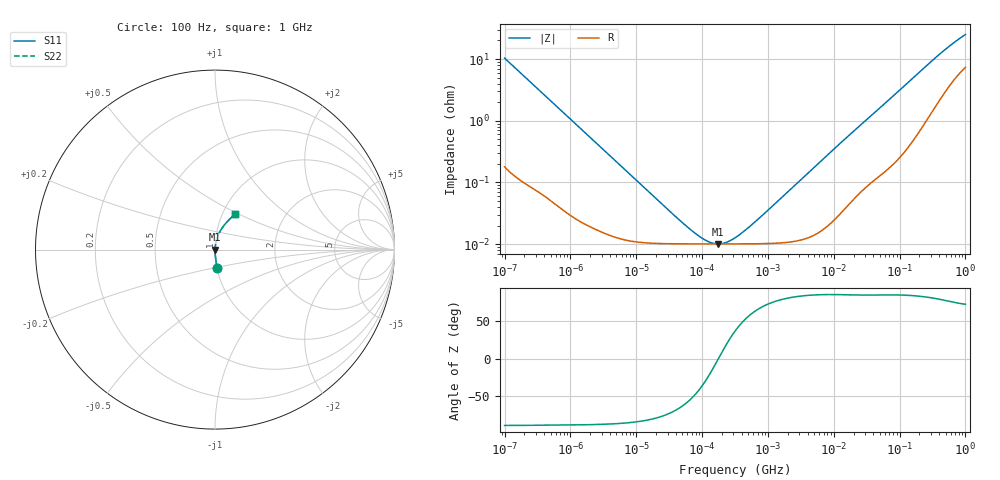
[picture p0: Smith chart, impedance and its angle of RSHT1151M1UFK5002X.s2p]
! RSHT1151M1UFK5002X  S-PARAMETER MODEL  (General Type)
! Model Generated by ELNA Corporation (http://www.ty-top.com)
! Version 1.0
! ELNA Control No.201201
! Copyright (c) 2020 ELNA CO.,LTD. All Rights Reserved.
! Products Name : CONDUCTIVE POLYMER HYBRID ALUMINUM ELECTROLYTIC CAPACITORS
! Characteristics :
!  Capacitance  :  150uF  ,  Rated voltage  :  50V
!  Operating Temp. Range  :  -55 to +105 degC  ,  Endurance  :  5000hr at 105 degC
!  Dimension D  :  10mm  ,  Dimension L  :  12.5mm
! Frequency Range : 100Hz - 1GHz
! External Node Assignments :
!  1  o---| |---o  2
# MHz S RI R 50
!Freq[MHz].  S11 Real  S11 Imag  S21 Real  S21 Imag  S12 Real  S12 Imag  S22 Real  S22 Imag
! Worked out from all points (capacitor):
!   401 points, 100 Hz to 1 GHz, reference 50 ohm
!   read as one part in series: C = 153 uF near 108 Hz
!   lowest |Z| = 10.1 mohm at 172.8 kHz (marker M1)
!   series resonance near 176.2 kHz, so ESL is about 5.3 nH
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0.0001  0.0124 -0.1021  0.9876 0.1021  0.9876 0.1021  0.0124 -0.1021
0.000113  0.0099 -0.0908  0.9901 0.0908  0.9901 0.0908  0.0099 -0.0908
0.000183  0.00424 -0.0565  0.9958 0.0565  0.9958 0.0565  0.00424 -0.0565
0.000309  0.00187 -0.0337  0.9981 0.0337  0.9981 0.0337  0.00187 -0.0337
0.001488  0.000276 -0.00717  0.9997 0.00717  0.9997 0.00717  0.000276 -0.00717
0.022131  0.000103 -0.000484  0.9999 0.000484  0.9999 0.000484  0.000103 -0.000484
0.051582  0.000101 -0.000193  0.9999 0.000193  0.9999 0.000193  0.000101 -0.000193
0.087096  0.000101 -9.44e-05  0.9999 9.44e-05  0.9999 9.44e-05  0.000101 -9.44e-05
0.12517  0.000101 -4.31e-05  0.9999 4.31e-05  0.9999 4.31e-05  0.000101 -4.31e-05
0.147062  0.000101 -2.24e-05  0.9999 2.24e-05  0.9999 2.24e-05  0.000101 -2.24e-05
0.172783  0.000101 -2.41e-06  0.9999 2.41e-06  0.9999 2.41e-06  0.000101 -2.41e-06
0.229087  0.000101 3.28e-05  0.9999 -3.28e-05  0.9999 -3.28e-05  0.000101 3.28e-05
0.316228  0.000101 7.64e-05  0.9999 -7.64e-05  0.9999 -7.64e-05  0.000101 7.64e-05
0.436516  0.000101 0.000128  0.9999 -0.000128  0.9999 -0.000128  0.000101 0.000128
0.679986  0.000102 0.000222  0.9999 -0.000222  0.9999 -0.000222  0.000102 0.000222
4.704354  0.000138 0.00164  0.9999 -0.00164  0.9999 -0.00164  0.000138 0.00164
13.96368  0.000374 0.00478  0.9996 -0.00478  0.9996 -0.00478  0.000374 0.00478
69.9842  0.00221 0.022  0.9978 -0.022  0.9978 -0.022  0.00221 0.022
169.8244  0.00784 0.0517  0.9922 -0.0517  0.9922 -0.0517  0.00784 0.0517
380.1894  0.0306 0.1061  0.9694 -0.1061  0.9694 -0.1061  0.0306 0.1061
641.9482  0.0671 0.1547  0.9329 -0.1547  0.9329 -0.1547  0.0671 0.1547
1000  0.1123 0.1981  0.8877 -0.1981  0.8877 -0.1981  0.1123 0.1981
